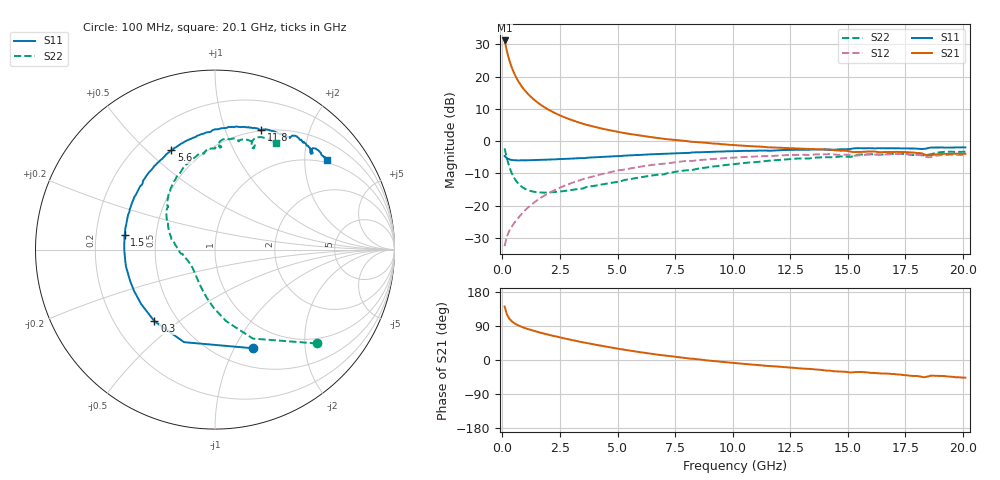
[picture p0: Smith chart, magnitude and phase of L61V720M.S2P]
!  Infineon Technologies AG
! BFR380L3 , PF131585-7, No.6, Th 09.10.01, soldered on pcb-board, measured with PP GSG850
!  Vce=1.75 V,  Ic=20.0 mA
! Common Emitter S-Parameters:  15. November 2001
#  GHz  S  MA  R  50
! f  S11  S21  S12  S22
! GHz  Mag  Ang  Mag  Ang  Mag  Ang  Mag  Ang
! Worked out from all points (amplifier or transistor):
!   201 points, 100 MHz to 20.1 GHz, reference 50 ohm
!   highest |S21| = 31.2 dB at 100 MHz (marker M1)
!   |S21| within 3 dB of that: start of sweep to 191.5 MHz
!   unconditionally stable (mu >= 1): 1.377 GHz to 4.46 GHz
!   at 3.4 GHz: K = 1.02, MAG = 8.0 dB, |S12| = -12.0 dB
!   at 10.1 GHz: K = 0.96, MSG = 1.9 dB, |S12| = -5.1 dB
!   at 20.1 GHz: K = 0.99, MSG = 0.1 dB, |S12| = -4.2 dB
!   S11 on the Smith chart (normalised r, x): 100 MHz: 0.71, -1.19; 300 MHz: 0.37, -0.41; 1.5 GHz: 0.33, +0.07; 5.6 GHz: 0.34, +0.60; 11.8 GHz: 0.49, +1.34; 20.1 GHz: 0.92, +2.55
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0.1  0.589 -69.0  36.26 141.2  0.02362 62.3  0.7721 -42.6
0.2  0.5438 -108.5  24.86 120.3  0.03343 53.8  0.5389 -66.9
0.3  0.5227 -130.3  18.17 109.6  0.04061 53.3  0.4036 -81.1
0.4  0.5111 -143.6  14.15 102.8  0.0467 54.6  0.3244 -91.3
0.5  0.5065 -152.6  11.55 97.9  0.05285 56.4  0.2748 -99.2
0.6  0.5043 -159.6  9.721 94.3  0.05903 58.2  0.242 -105.8
0.7  0.5029 -165.1  8.407 91.1  0.06543 59.6  0.219 -111.6
0.8  0.5049 -169.2  7.395 88.5  0.07198 60.8  0.2026 -116.6
1  0.504 -176.3  5.971 83.9  0.08563 62.4  0.1816 -125.2
1.2  0.506 178.0  5.009 80.0  0.09945 63.1  0.1702 -132.2
1.5  0.5103 171.0  4.045 74.7  0.1205 63.4  0.1615 -140.7
1.9  0.5151 163.1  3.234 68.3  0.1486 62.5  0.1594 -149.6
2.3  0.5215 156.1  2.707 62.5  0.1764 60.9  0.1629 -157.1
2.9  0.5365 146.9  2.193 54.3  0.2175 57.8  0.1729 -166.2
3.5  0.5446 138.3  1.857 46.6  0.2578 54.1  0.1846 -172.8
5.6  0.6044 113.7  1.284 24.3  0.381 40.0  0.2601 162.6
6.8  0.6319 102.0  1.111 13.5  0.4419 31.4  0.3026 149.5
10.1  0.6982 78.0  0.8682 -8.1  0.5567 10.1  0.4424 121.2
11.8  0.7152 68.9  0.7977 -16.4  0.5928 0.1  0.5037 107.3
13.5  0.7379 60.6  0.7546 -24.3  0.6182 -10.1  0.5488 95.8
16.8  0.7747 48.4  0.6804 -36.0  0.6237 -25.7  0.6327 75.9
20.1  0.7986 38.8  0.6384 -46.5  0.6178 -39.1  0.6864 60.3
